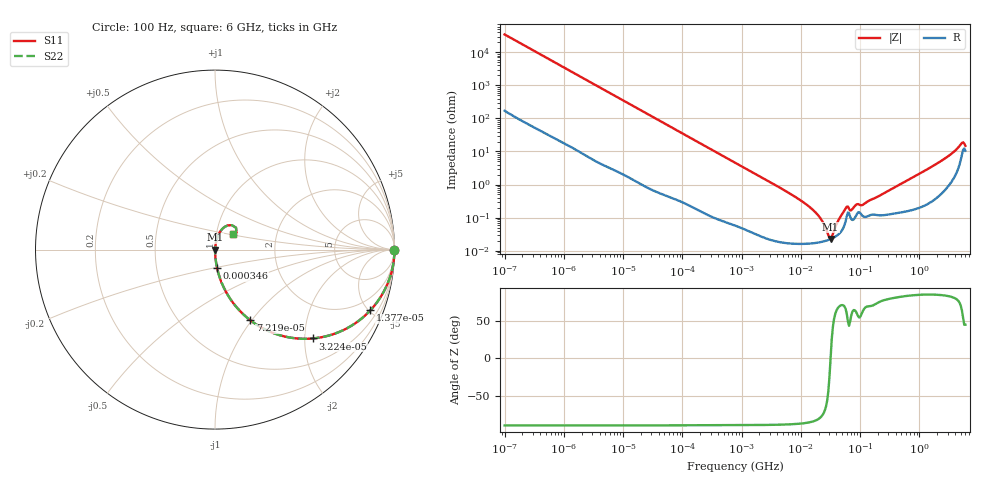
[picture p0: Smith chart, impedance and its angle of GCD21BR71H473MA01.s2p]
!Murata Part Number: GCD21BR71H473MA01
!These Parameters are Measured in Series Mode Connection
!Data Generated on Jan 08, 2026
!  o--ll--o
!Port1  Port2
!  o------o
!Operation Temp=25[degC], DC Bias Voltage=0[V]
!Freq. Start=100[Hz] Stop=6[GHz] 401[Steps]
# Hz S RI R 50
!Freq.(Hz) S11(Real) S11(Imag) S21(Real) S21(Imag) S12(Real) S12(Imag) S22(Real) S22(Imag)
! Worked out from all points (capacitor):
!   401 points, 100 Hz to 6 GHz, reference 50 ohm
!   read as one part in series: C = 45.8 nF near 109 Hz
!   lowest |Z| = 22.4 mohm at 31.85 MHz (marker M1)
!   series resonance near 31.78 MHz, so ESL is about 550 pH
!   S11 on the Smith chart (normalised r, x): 100 Hz: open; 13.77 kHz: 1.03, -5.12; 32.24 kHz: 1.01, -2.19; 72.19 kHz: 1.01, -0.98; 346 kHz: 1.00, -0.21; 6 GHz: 1.21, +0.21
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100  1 -0.00288  2.25e-05 0.00288  2.25e-05 0.00288  1 -0.00288
2008  0.9964 -0.0571  0.00356 0.0571  0.00356 0.0571  0.9964 -0.0571
13772  0.8662 -0.3376  0.1338 0.3376  0.1338 0.3376  0.8662 -0.3376
32244  0.5457 -0.4949  0.4543 0.4949  0.4543 0.4949  0.5457 -0.4949
40335  0.4352 -0.4926  0.5648 0.4926  0.5648 0.4926  0.4352 -0.4926
72189  0.1962 -0.3934  0.8038 0.3934  0.8038 0.3934  0.1962 -0.3934
135116  0.0667 -0.2453  0.9333 0.2453  0.9333 0.2453  0.0667 -0.2453
345986  0.0115 -0.102  0.9885 0.102  0.9885 0.102  0.0115 -0.102
774597  0.00271 -0.0462  0.9973 0.0462  0.9973 0.0462  0.00271 -0.0462
6644369  0.000191 -0.00523  0.9998 0.00523  0.9998 0.00523  0.000191 -0.00523
1.555665e7  0.000169 -0.00179  0.9998 0.00179  0.9998 0.00179  0.000169 -0.00179
2.128304e7  0.000181 -0.000952  0.9998 0.000952  0.9998 0.000952  0.000181 -0.000952
2.911731e7  0.00021 -0.000205  0.9998 0.000205  0.9998 0.000205  0.00021 -0.000205
3.184506e7  0.000223 5.1e-06  0.9998 -5.1e-06  0.9998 -5.1e-06  0.000223 5.1e-06
5.699437e7  0.00077 0.00173  0.9992 -0.00173  0.9992 -0.00173  0.00077 0.00173
7.129496e7  0.000891 0.00141  0.9991 -0.00141  0.9991 -0.00141  0.000891 0.00141
8.918374e7  0.00131 0.00217  0.9987 -0.00217  0.9987 -0.00217  0.00131 0.00217
1.115611e8  0.00111 0.00217  0.9989 -0.00217  0.9989 -0.00217  0.00111 0.00217
3.124326e8  0.00129 0.00657  0.9987 -0.00657  0.9987 -0.00657  0.00129 0.00657
2.240541e9  0.00714 0.0485  0.9929 -0.0485  0.9929 -0.0485  0.00714 0.0485
5.016141e9  0.0729 0.1352  0.9271 -0.1352  0.9271 -0.1352  0.0729 0.1352
6e9  0.1029 0.0845  0.8971 -0.0845  0.8971 -0.0845  0.1029 0.0845
